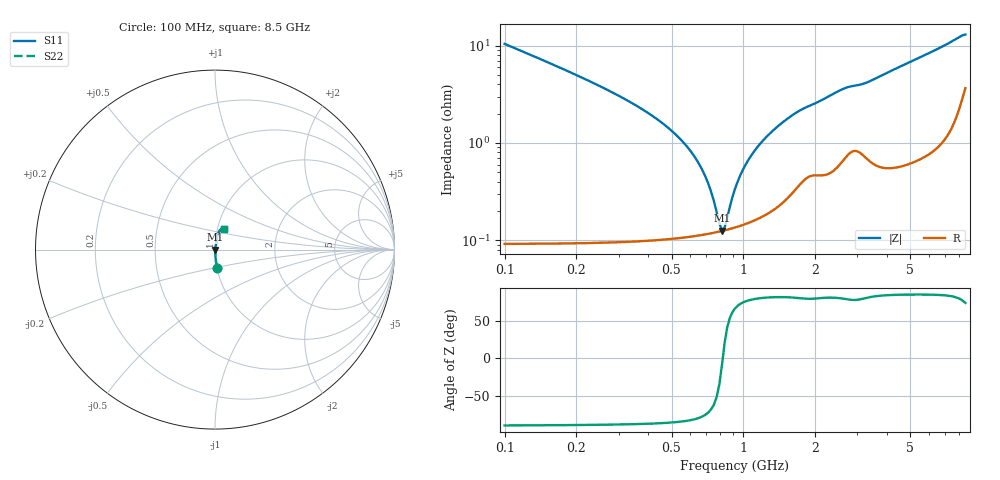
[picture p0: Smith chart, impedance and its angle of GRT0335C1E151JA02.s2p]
!Murata Part Number: GRT0335C1E151JA02
!These Parameters are Measured in Series Mode Connection
!Data Generated on Jun 19, 2026
!  o--ll--o
!Port1  Port2
!  o------o
!Operation Temp=25[degC], DC Bias Voltage=0[V]
!Freq. Start=100[MHz] Stop=9[GHz] 401[Steps]
# Hz S RI R 50
!Freq.(Hz) S11(Real) S11(Imag) S21(Real) S21(Imag) S12(Real) S12(Imag) S22(Real) S22(Imag)
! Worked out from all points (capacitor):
!   401 points, 100 MHz to 8.5 GHz, reference 50 ohm
!   read as one part in series: C = 150 pF near 142 MHz
!   lowest |Z| = 126 mohm at 814 MHz (marker M1)
!   series resonance near 819.2 MHz, so ESL is about 250 pH
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1e8  0.0117 -0.1032  0.9883 0.1032  0.9883 0.1032  0.0117 -0.1032
2.47e8  0.00246 -0.0389  0.9975 0.0389  0.9975 0.0389  0.00246 -0.0389
5.2e8  0.00119 -0.0122  0.9988 0.0122  0.9988 0.0122  0.00119 -0.0122
6.04e8  0.00115 -0.00802  0.9988 0.00802  0.9988 0.00802  0.00115 -0.00802
6.88e8  0.00116 -0.00455  0.9988 0.00455  0.9988 0.00455  0.00116 -0.00455
7.72e8  0.00121 -0.00154  0.9988 0.00154  0.9988 0.00154  0.00121 -0.00154
7.93e8  0.00123 -0.000844  0.9988 0.000844  0.9988 0.000844  0.00123 -0.000844
8.14e8  0.00124 -0.000165  0.9988 0.000165  0.9988 0.000165  0.00124 -0.000165
8.35e8  0.00126 0.000497  0.9987 -0.000497  0.9987 -0.000497  0.00126 0.000497
8.56e8  0.00128 0.00114  0.9987 -0.00114  0.9987 -0.00114  0.00128 0.00114
9.19e8  0.00136 0.003  0.9986 -0.003  0.9986 -0.003  0.00136 0.003
9.61e8  0.00141 0.00418  0.9986 -0.00418  0.9986 -0.00418  0.00141 0.00418
1.066e9  0.00158 0.00695  0.9984 -0.00695  0.9984 -0.00695  0.00158 0.00695
1.255e9  0.00199 0.0115  0.998 -0.0115  0.998 -0.0115  0.00199 0.0115
1.507e9  0.00289 0.017  0.9971 -0.017  0.9971 -0.017  0.00289 0.017
1.78e9  0.00453 0.022  0.9955 -0.022  0.9955 -0.022  0.00453 0.022
2.347e9  0.00596 0.0307  0.994 -0.0307  0.994 -0.0307  0.00596 0.0307
2.914e9  0.00962 0.0372  0.9904 -0.0372  0.9904 -0.0372  0.00962 0.0372
4.3e9  0.00874 0.0564  0.9913 -0.0564  0.9913 -0.0564  0.00874 0.0564
5.707e9  0.0132 0.0776  0.9868 -0.0776  0.9868 -0.0776  0.0132 0.0776
7.114e9  0.0217 0.0999  0.9783 -0.0999  0.9783 -0.0999  0.0217 0.0999
8.5e9  0.0492 0.1149  0.9508 -0.1149  0.9508 -0.1149  0.0492 0.1149
